ORGANIZATION_BLOCK OB 100
BEGIN
	L		MD 0
	__ASSERT==	__ACCU 1,	0
	L		100
	T		MD 0
END_ORGANIZATION_BLOCK



ORGANIZATION_BLOCK OB 101
BEGIN
	L		MD 0
	__ASSERT==	__ACCU 1,	0
	L		101
	T		MD 0
END_ORGANIZATION_BLOCK



ORGANIZATION_BLOCK OB 102
BEGIN
	L		MD 0
	__ASSERT==	__ACCU 1,	0
	L		102
	T		MD 0
END_ORGANIZATION_BLOCK



ORGANIZATION_BLOCK OB 1
BEGIN
	// assert 2-accus
	__FEATURE	0
	__ASSERT==	__ACCU 1,	2


	// check that OB 100 was executed
	L		MD 0
	__ASSERT==	__ACCU 1,	100


	CALL SFC 46 // STOP CPU
END_ORGANIZATION_BLOCK
